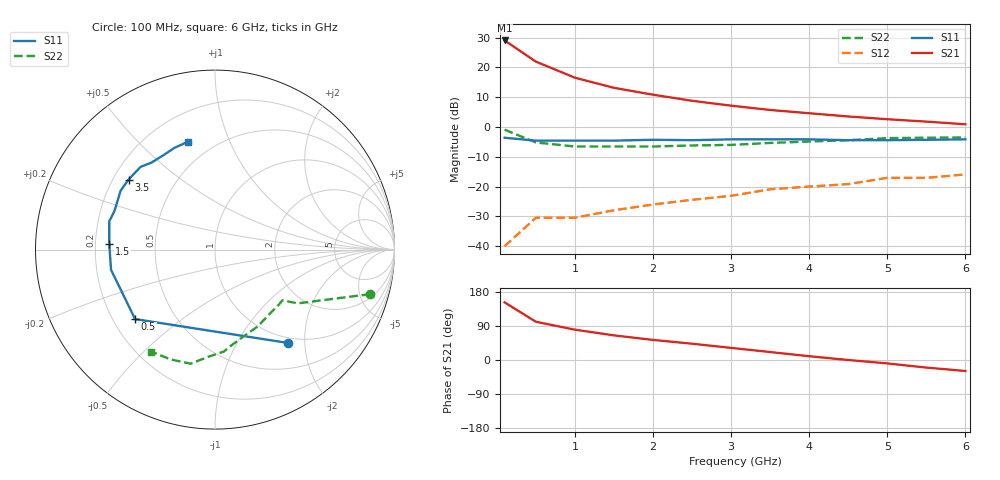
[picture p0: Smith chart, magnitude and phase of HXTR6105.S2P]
! HXTR-6105 Common Emitter
! Vce=15V  Ic=15mA
# ghz s ma r 50
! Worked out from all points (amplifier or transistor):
!   13 points, 100 MHz to 6 GHz, reference 50 ohm
!   highest |S21| = 29.0 dB at 100 MHz (marker M1)
!   |S21| within 3 dB of that: start of sweep to 269.1 MHz
!   unconditionally stable (mu >= 1): 914.2 MHz to 3.615 GHz
!   at 1 GHz: K = 1.12, MAG = 21.4 dB, |S12| = -30.5 dB
!   at 3 GHz: K = 1.22, MAG = 12.3 dB, |S12| = -23.1 dB
!   at 6 GHz: K = 0.65, MSG = 8.4 dB, |S12| = -15.9 dB
!   S11 on the Smith chart (normalised r, x): 100 MHz: 0.91, -1.67; 500 MHz: 0.29, -0.35; 1.5 GHz: 0.26, +0.02; 3.5 GHz: 0.26, +0.33; 6 GHz: 0.37, +0.71
0.1  0.66 -52.0  28.3 152.0  0.01 69.0  0.9 -16.0
0.5  0.59 -139.0  12.5 101.0  0.03 41.0  0.55 -33.0
1  0.59 -169.0  6.71 80.0  0.03 45.0  0.47 -37.0
1.5  0.59 177.0  4.54 65.0  0.04 49.0  0.47 -41.0
2  0.61 165.0  3.48 53.0  0.05 50.0  0.47 -50.0
2.5  0.6 159.0  2.75 43.0  0.06 51.0  0.49 -61.0
3  0.62 148.0  2.28 32.0  0.07 52.0  0.5 -68.0
3.5  0.62 141.0  1.93 21.0  0.09 49.0  0.54 -80.0
4  0.62 132.0  1.7 10.0  0.1 47.0  0.57 -85.0
4.5  0.6 126.0  1.5 0.0  0.11 45.0  0.6 -94.0
5  0.6 118.0  1.35 -9.0  0.14 42.0  0.65 -102.0
5.5  0.61 112.0  1.23 -20.0  0.14 35.0  0.66 -112.0
6  0.62 104.0  1.11 -29.0  0.16 31.0  0.67 -122.0
